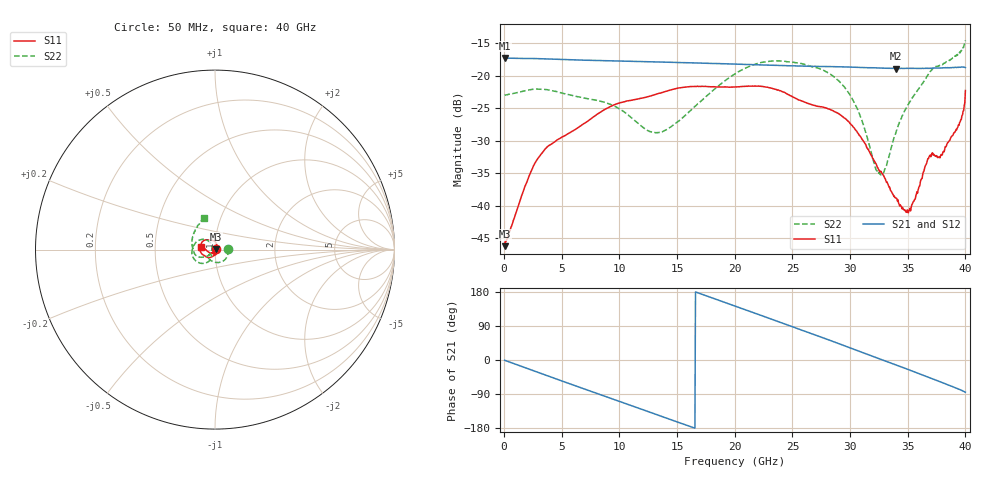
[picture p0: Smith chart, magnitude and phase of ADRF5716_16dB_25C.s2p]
! Device: ADRF5716
! Description: 30GHz 2-Bit Digital Attenuator
! Frequency: 100 MHz – 30 GHz
! Ports:
! ATTIN  = Port 1
! ATTOUT = Port 2
! State: 16 dB Attenuation selected
! Supply Voltage:
! VDD  =  +3.30 Volts
! VSS  =  -3.30 Volts
! Control Voltages:
! D5 = 3.3V, D6 = 0V
! Temperature = +25 C
! Data: Data was collected using a calibrated network analyzer.
!  The reference plane is the package pins of ADRF5716 switch.
! Note: Analog Devices supplies this data as a sample of measured data for this product.
!  Your particular data for this product may vary.
!  Analog Devices reserves the right to change this data at anytime
# HZ S DB R 50
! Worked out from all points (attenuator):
!   800 points, 50 MHz to 40 GHz, reference 50 ohm
!   highest |S21| = -17.26 dB at 100 MHz (marker M1); lowest = -18.9 dB at 33.95 GHz (marker M2)
!   lowest |S11| = -46.2 dB at 50 MHz (marker M3), VSWR 1.01, Z = 50.5 + j0.0973 ohm
!   |S11| at or under -10 dB: start of sweep to end of sweep
!   |S22| runs from -35.2 to -14.6 dB; largest |S21 - S12| = 0
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5e7  -46.19 11.3  -17.27 -0.6  -17.27 -0.6  -23.01 0.7
1e8  -45.47 4.0  -17.26 -1.2  -17.26 -1.2  -22.93 -0.6
2.85e9  -32.91 -63.3  -17.35 -31.6  -17.35 -31.6  -22.03 -43.0
6.75e9  -27.54 -111.7  -17.58 -74.1  -17.58 -74.1  -23.32 -98.5
9.6e9  -24.41 -133.4  -17.71 -104.9  -17.71 -104.9  -24.68 -128.5
1.34e10  -22.69 -157.3  -17.87 -145.9  -17.87 -145.9  -28.73 -127.7
2.005e10  -21.70 163.3  -18.19 141.9  -18.19 141.9  -19.66 -132.0
2.3e10  -21.82 143.2  -18.35 109.9  -18.35 109.9  -17.76 -160.7
2.67e10  -24.45 120.7  -18.54 69.1  -18.54 69.1  -18.58 165.5
2.85e10  -25.35 106.5  -18.58 49.1  -18.58 49.1  -19.99 147.0
2.995e10  -27.18 88.5  -18.64 32.7  -18.64 32.7  -22.80 131.8
3.095e10  -29.44 76.2  -18.71 21.2  -18.71 21.2  -26.50 124.4
3.245e10  -34.32 60.9  -18.78 4.2  -18.78 4.2  -35.02 163.6
3.285e10  -35.21 57.1  -18.81 -0.4  -18.81 -0.4  -34.98 -172.3
3.335e10  -37.01 48.2  -18.84 -5.9  -18.84 -5.9  -32.56 -147.1
3.395e10  -38.77 37.2  -18.88 -12.6  -18.88 -12.6  -28.88 -137.4
3.47e10  -40.66 6.1  -18.85 -21.1  -18.85 -21.1  -25.46 -138.8
3.52e10  -40.36 -19.1  -18.85 -26.8  -18.85 -26.8  -23.94 -142.2
3.69e10  -32.29 -101.0  -18.84 -46.7  -18.84 -46.7  -19.50 -159.6
3.78e10  -32.60 -128.7  -18.80 -57.3  -18.80 -57.3  -18.39 -178.9
3.935e10  -27.86 -162.2  -18.70 -76.0  -18.70 -76.0  -16.76 145.4
4e10  -22.25 167.5  -18.74 -85.0  -18.74 -85.0  -14.56 109.2
